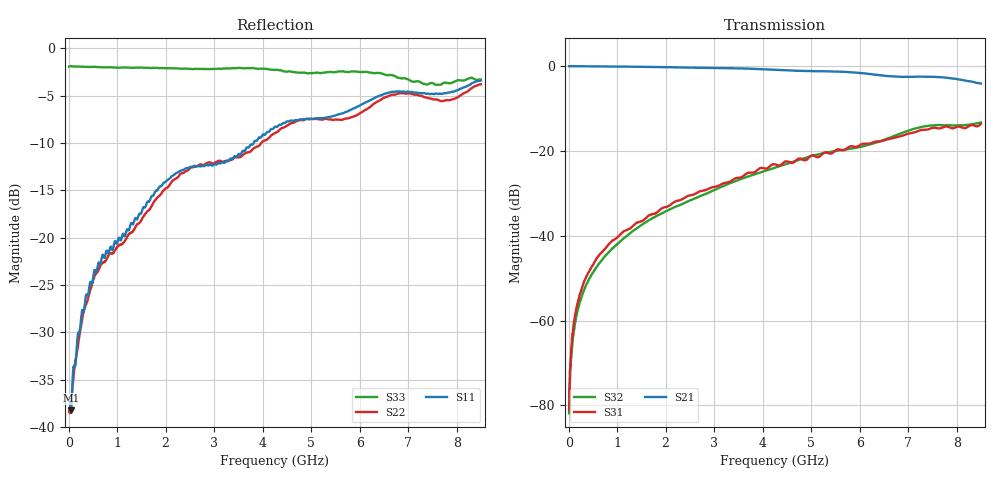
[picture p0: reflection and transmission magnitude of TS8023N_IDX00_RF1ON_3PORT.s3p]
!Created with skrf (http://scikit-rf.org).
# GHz S RI R 50.0
!freq ReS11 ImS11 ReS12 ImS12 ReS13 ImS13
! ReS21 ImS21 ReS22 ImS22 ReS23 ImS23
! ReS31 ImS31 ReS32 ImS32 ReS33 ImS33
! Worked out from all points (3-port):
!   1601 points, 10 MHz to 8.5 GHz, reference 50 ohm
!   strongest paths, dB at 10 MHz, 2.132 GHz, 4.255 GHz, 6.378 GHz, 8.5 GHz:
!     S21: -0.1, -0.4, -1.0, -2.2, -4.2
!     S31: -81.1, -32.5, -23.3, -17.8, -13.7
!     S32: -81.8, -33.6, -24.0, -18.0, -13.4
!   lowest |S11| = -38.3 dB at 41.84 MHz (marker M1), VSWR 1.02, Z = 51 - j0.717 ohm
!   |S11| at or under -10 dB: start of sweep to 3.814 GHz
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0.01  0.0139 -0.00016  0.9835 -0.00318  2.8e-05 8.47e-05
      0.9834 -0.00344  0.0125 0.000144  3.87e-05 9.49e-05
      3.3e-05 8.14e-05  4.61e-05 6.64e-05  -0.8022 0.00247
0.0418375  0.00998 -0.00703  0.9832 -0.0132  2.48e-05 0.000383
           0.983 -0.0129  0.011 -0.00549  3.49e-05 0.000296
           5.19e-05 0.000351  3.21e-05 0.000293  -0.8057 0.00652
0.116125  0.01 -0.0184  0.9814 -0.035  2.36e-05 0.00101
          0.9814 -0.0351  0.0101 -0.0177  2.44e-05 0.000808
          2.43e-05 0.001  7.68e-06 0.000779  -0.8036 0.0185
0.2647  0.012 -0.037  0.9772 -0.0788  -9.83e-05 0.00232
        0.9772 -0.079  0.00629 -0.0347  -4.27e-05 0.00188
        -8.75e-05 0.00233  -5.59e-05 0.00188  -0.7993 0.0397
0.8696125  -0.00401 -0.0896  0.9419 -0.2494  -0.000542 0.00833
           0.942 -0.2492  -0.0219 -0.0796  -0.000388 0.00671
           -0.000522 0.00836  -0.000397 0.00672  -0.7783 0.1606
2.312912  -0.1143 -0.1948  0.7337 -0.6023  8.03e-05 0.0263
          0.7345 -0.6025  -0.1386 -0.1684  0.00258 0.0229
          0.000113 0.0263  0.0026 0.0229  -0.6807 0.3843
4.255  -0.3375 -0.1861  0.261 -0.852  0.0224 0.065
       0.2603 -0.8512  -0.355 -0.0325  0.0314 0.0543
       0.0223 0.0649  0.0316 0.0544  -0.434 0.6364
6.839144  -0.5778 0.1284  -0.3213 -0.6623  0.1153 0.0912
          -0.3209 -0.6627  -0.4249 0.3946  0.1507 0.0486
          0.1152 0.0912  0.1508 0.0486  -0.0194 0.6962
7.953456  -0.4882 0.336  -0.5023 -0.4863  0.1768 0.052
          -0.5037 -0.4873  -0.1641 0.5163  0.1919 -0.0465
          0.1773 0.0521  0.192 -0.0463  0.3401 0.5747
8.5  -0.4787 0.479  -0.5039 -0.3507  0.1996 0.0504
     -0.5043 -0.3515  -0.0723 0.642  0.2038 -0.0654
     0.1997 0.0506  0.2038 -0.0655  0.3216 0.6053
